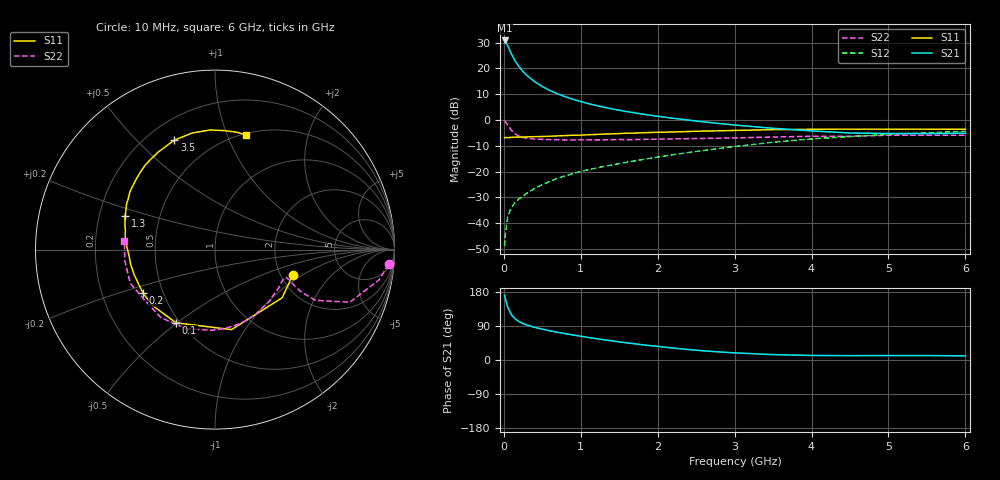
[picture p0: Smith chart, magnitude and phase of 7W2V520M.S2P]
! Infineon Technologies  Discrete & RF Semiconductors
! BFS17W
! Si NPN RF Bipolar Junction Transistor in SOT323
! VCE = 2.5 V  IC = 20 mA
! Common Emitter S-Parameters:  August  1999
# GHz  S  MA  R  50
!  f  S11  S21  S12  S22
! GHz  MAG  ANG  MAG  ANG  MAG  ANG  MAG  ANG
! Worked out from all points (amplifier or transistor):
!   36 points, 10 MHz to 6 GHz, reference 50 ohm
!   highest |S21| = 30.8 dB at 10 MHz (marker M1)
!   |S21| within 3 dB of that: start of sweep to 65.08 MHz
!   unconditionally stable (mu >= 1): 249 MHz to 2.487 GHz; 4.264 GHz to end of sweep
!   at 250 MHz: K = 1.00, MAG = 23.8 dB, |S12| = -29.4 dB
!   at 1.4 GHz: K = 1.21, MAG = 8.1 dB, |S12| = -17.4 dB
!   at 6 GHz: K = 1.08, MAG = -2.1 dB, |S12| = -4.4 dB
!   S11 on the Smith chart (normalised r, x): 10 MHz: 2.31, -0.84; 100 MHz: 0.48, -0.50; 200 MHz: 0.39, -0.24; 1.3 GHz: 0.31, +0.16; 3.5 GHz: 0.31, +0.65; 6 GHz: 0.52, +1.17
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0.01  0.4558 -18.3  34.8 171.0  0.0036 81.1  0.9704 -4.9
0.02  0.4604 -35.7  33.77 161.7  0.006 81.7  0.9301 -10.4
0.05  0.4552 -78.4  27.66 139.8  0.0137 67.0  0.8066 -21.3
0.1  0.462 -118.0  18.84 119.1  0.0206 57.4  0.6269 -26.8
0.15  0.4664 -137.9  13.69 107.9  0.0254 57.0  0.5328 -26.1
0.2  0.4687 -148.8  10.67 101.1  0.0299 59.4  0.4875 -24.5
0.25  0.4673 -156.6  8.678 96.1  0.0337 60.6  0.4605 -22.9
0.3  0.4708 -162.0  7.299 92.3  0.0384 63.2  0.4461 -22.2
0.4  0.477 -169.7  5.541 86.1  0.0471 65.0  0.4279 -21.5
0.5  0.4793 -174.9  4.459 81.3  0.056 67.4  0.4219 -21.7
0.6  0.4851 -179.0  3.719 77.0  0.0649 68.5  0.4175 -22.8
0.7  0.4931 177.5  3.211 73.1  0.0746 69.0  0.4141 -24.4
0.9  0.5073 170.9  2.516 66.0  0.0916 69.3  0.4115 -28.4
1.1  0.5188 165.2  2.077 59.3  0.1093 69.6  0.4131 -33.3
1.3  0.5345 159.6  1.771 53.4  0.1266 69.7  0.4127 -38.9
1.7  0.5583 150.2  1.379 42.8  0.1617 70.0  0.4179 -50.7
2.2  0.5877 138.6  1.082 31.5  0.2125 69.3  0.4314 -66.7
2.8  0.6185 124.9  0.856 21.3  0.2813 65.7  0.4444 -86.7
3.5  0.651 110.3  0.691 14.2  0.3713 59.0  0.4689 -110.2
4.5  0.667 92.4  0.561 11.5  0.4783 45.9  0.4827 -144.3
5.5  0.6652 79.6  0.545 11.7  0.5663 33.4  0.5065 -172.8
6  0.6616 74.7  0.556 11.0  0.6012 27.4  0.5065 174.7
